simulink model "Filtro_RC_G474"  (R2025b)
settings: Solver=FixedStepAuto  StartTime=0.0  StopTime=inf  RelTol=1e-3  EnableMultiTasking=on
libraries: stm32f4xxblockslib x2, slpidlib x1

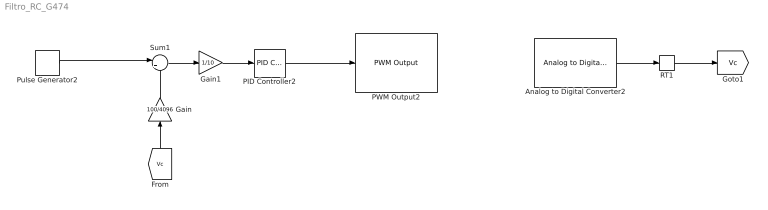
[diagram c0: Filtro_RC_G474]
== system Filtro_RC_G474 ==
  Analog to Digital Converter2 : stm32f4xxblockslib/Analog to Digital Converter  ADCModule=ADC3  ConversionGroup=Injected  TriggerMode=Read results only  NumberOfConversions=1  EnableBufferConv=off  BufferLength=1  OutputStatus=off  SampleTime=-1  EnableSimPort=off  hoistedMaskSrc=ECSoC/ECSimCodegen/Analog to Digital Converter
  Gain : Gain  Gain=100/4096
  Gain1 : Gain  Gain=1/10
  PID Controller2 : slpidlib/PID Controller  Controller=PI  Form=Parallel  TimeDomain=Discrete-time  UseExternalTs=off  SampleTime=-1  IntegratorMethod=Forward Euler  FilterMethod=Forward Euler  ControllerParametersSource=internal  P=15  I=1500  UseKiTs=off  D=0  UseExternalDerivativeSource=off  N=0  UseFilter=on  TunerSelectOption=Transfer Function Based (PID Tuner App)  InitialConditionSource=internal  InitialConditionForIntegrator=0  InitialConditionForFilter=0  DifferentiatorICPrevScaledInput=0  ExternalReset=none  TrackingMode=off  Kt=1  LimitOutput=on  SatLimitsSource=internal  UpperSaturationLimit=100  LowerSaturationLimit=0  LinearizeAsGain=on  AntiWindupMode=clamping  Kb=1  LimitIntegrator=off  UpperIntegratorSaturationLimit=inf  LowerIntegratorSaturationLimit=-inf  POutMin=[]  POutMax=[]  IOutMin=[]  IOutMax=[]  DOutMin=[]  DOutMax=[]  NOutMin=[]  NOutMax=[]  SumOutMin=[]  SumOutMax=[]  SaturationOutMin=[]  SaturationOutMax=[]  PParamMin=[]  PParamMax=[]  IParamMin=[]  IParamMax=[]  DParamMin=[]  DParamMax=[]  NParamMin=[]  NParamMax=[]  KbParamMin=[]  KbParamMax=[]  KtParamMin=[]  KtParamMax=[]  KbOutMin=[]  KbOutMax=[]  KtOutMin=[]  KtOutMax=[]  IntegratorOutMin=[]  IntegratorOutMax=[]  FilterOutMin=[]  FilterOutMax=[]  SumI1OutMin=[]  SumI1OutMax=[]  SumI2OutMin=[]  SumI2OutMax=[]  SumI3OutMin=[]  SumI3OutMax=[]  SumI4OutMin=[]  SumI4OutMax=[]  SumDOutMin=[]  SumDOutMax=[]  DifferentiatorOutMin=[]  DifferentiatorOutMax=[]  FilterDiffOutCoefMin=[]  FilterDiffOutCoefMax=[]  ReciprocalOutMin=[]  ReciprocalOutMax=[]  SumDenOutMin=[]  SumDenOutMax=[]  SumNumOutMin=[]  SumNumOutMax=[]  DivideOutMin=[]  DivideOutMax=[]  UdiffTsProdOutMin=[]  UdiffTsProdOutMax=[]  NTsProdOutMin=[]  NTsProdOutMax=[]  UintegralTsProdOutMin=[]  UintegralTsProdOutMax=[]  UngainTsProdOutMin=[]  UngainTsProdOutMax=[]  ClampingZeroOutDataTypeStr=Inherit: Inherit via back propagation  ClampingZeroOutMin=[]  ClampingZeroOutMax=[]  FilterDenConstantOutDataTypeStr=Inherit: Inherit via back propagation  FilterDenConstantOutMin=[]  FilterDenConstantOutMax=[]  PCopyOutDataTypeStr=Inherit: Inherit via back propagation  PCopyOutMin=[]  PCopyOutMax=[]  NCopyOutDataTypeStr=Inherit: Inherit via back propagation  NCopyOutMin=[]  NCopyOutMax=[]  IntegratorContinuousStateAttributes=''  IntegratorStateMustResolveToSignalObject=off  IntegratorRTWStateStorageClass=Auto  FilterContinuousStateAttributes=''  FilterStateMustResolveToSignalObject=off  FilterRTWStateStorageClass=Auto  ParallelPVariant=InternalParameters  IdealPVariant=Disabled  IVariant=InternalParameters  DVariant=Disabled  IntegratorVariant=Discrete  SatVariant=Enabled  AWVariant=DiscClampingParallel  PCopyVariant=Disabled  TRVariant=Disabled  FdbkBlocksVariant=Forward  IdealPFdbkVariant=Disabled  SatFdbkVariant=Disabled  DerivativeFilterVariant=Disabled  NVariant=Disabled  NCopyVariant=Disabled_SignalSpec  FilterICVariant=Disabled  IntegratorICVariant=InternalICs  ExternalResetVariant=Disabled  TRSumVariant=Passthrough  SumFdbkVariant=Disabled  SumVariant=Sum_PI  TsampFilterVariant=InternalTs  TsampNgainVariant=Passthrough  TsampIntegralVariant=Disabled_SignalSpec  ExternalSaturationOutDataTypeStr=Inherit: Same as second input  DerivativeSourceVariant=Disabled  PreIntVariant=InternalPreInt
  PWM Output2 : stm32f4xxblockslib/PWM Output  ProcessorFamily=STM32G4  TimerModule=TIM3  DutycycleUnits=Percentage  EnableChannel1=off  EnableCaptureCompare1Input=off  EnableCaptureCompare1ComplementaryInput=off  EnableOutputCompare1ModeInput=off  EnableChannel2=on  EnableCaptureCompare2Input=off  EnableCaptureCompare2ComplementaryInput=off  EnableOutputCompare2ModeInput=off  EnableChannel3=off  EnableCaptureCompare3Input=off  EnableCaptureCompare3ComplementaryInput=off  EnableOutputCompare3ModeInput=off  EnableChannel4=off  EnableCaptureCompare4Input=off  EnableCaptureCompare4ComplementaryInput=off  EnableOutputCompare4ModeInput=off  EnableChannel5=off  EnableCaptureCompare5Input=off  EnableOutputCompare5ModeInput=off  EnableChannel6=off  EnableCaptureCompare6Input=off  EnableOutputCompare6ModeInput=off  EnableCounterInput=off  EnableMainOutputInput=off  EnableFrequencyInput=off  SetRCAfterCE=off  OutputDirection=off  OutputMainOutputEnableStatus=off  SampleTime=0.1  EnableSimPort=off  EnableUpdateEvent=off  EnableCaptureCompare1Event=off  EnableCaptureCompare2Event=off  EnableCaptureCompare3Event=off  EnableCaptureCompare4Event=off  EnableTriggerEvent=off  EnableBreakEvent=off  EnableBreakEvent2=off  hoistedMaskSrc=ECSoC/ECSimCodegen/PWM Output
  Pulse Generator2 : DiscretePulseGenerator  PulseType=Time based  Amplitude=90  Period=0.2  PulseWidth=50
  RT1 : RateTransition  Deterministic=off  OutPortSampleTime=0.0001
  Sum1 : Sum  Inputs=|+-
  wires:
  Pulse Generator2/1 -> Sum1/1
  RT1/1 -> [Vc]
  Analog to Digital Converter2/1 -> RT1/1
  Sum1/1 -> Gain1/1
  [Vc] -> Gain/1
  PID Controller2/1 -> PWM Output2/1
  Gain1/1 -> PID Controller2/1
  Gain/1 -> Sum1/2
